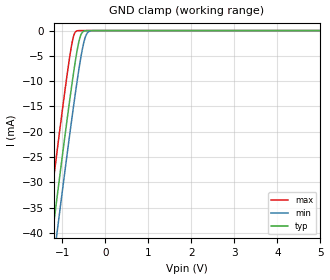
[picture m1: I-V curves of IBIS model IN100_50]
| TEXAS INSTRUMENTS INCORPORATED - Standard Linear and
|   Logic Group / High Volume Linear
| EMI Filter with Integrated VCC Clamp for SIM Card Interface
| Part#   VCC Voltage Range   Package-type   #pins
|TPD6F002QDSV   4.5 to 5.5V   QFN   13
[IBIS Ver]   3.2
[Comment char]  |_char
[File Name]   tpd6f002.ibs
[File Rev]   1.0 | A0
[Date]   December 10, 2014
[Source]   Data created from TI-SPICE simulations at TI-SLL/HVL.
   The following is an IBIS list for the TPD6F002.
   Please contact sllibis@ti.com with questions and
   comments concerning SLL IBIS models.
[Notes]   Revision History:
   1.0: 02/24/2011
   - Initial version of the model
   - This file contains package information for the SOT 8-pin
   (DSV) package as [Component] TPD6F002_DSV
   - This device can be powered at 5 volt Vcc
[Disclaimer]
| This model is designed as an aid for customers of Texas Instruments.
| TI and its licensors and suppliers make no warranties, either expressed
| or implied, with respect to this  model, including the warranties of
| merchantability or fitness for a particular purpose. The model is
| provided solely on an "as is" basis. The entire risk as to its quality
| and performance is with the customer.
[Copyright]
| (C) Copyright 2011 Texas Instruments Incorporated. All rights reserved.
| Component TPD6F002_DSV 13-PIN QFN
[Component]   TPD6F002_DSV
[Manufacturer]   Texas Instruments, Inc.
[Package]
|   typ   min   max
R_pkg   5.374e-02   1.500e-02   5.374e-02
L_pkg   6.554e-10   6.400e-12   7.112e-10
C_pkg   9.454e-14   5.280e-14   9.871e-14
[Pin]   signal_name   model_name   R_pin   L_pin   C_pin
1   Ch1_In   IN100_50   5.701e-02   7.112e-10   8.801e-14
2   Ch1_In   IN100_50   5.253e-02   6.367e-10   9.865e-14
3   Ch1_In   IN100_50   5.161e-02   6.235e-10   9.692e-14
4   Ch1_In   IN100_50   5.172e-02   6.216e-10   9.691e-14
5   Ch1_In   IN100_50   5.260e-02   6.372e-10   9.871e-14
6   Ch1_In   IN100_50   5.707e-02   7.096e-10   8.808e-14
7   Ch1_In   IN100_50   5.714e-02   7.049e-10   8.802e-14
8   Ch1_In   IN100_50   5.251e-02   6.347e-10   9.869e-14
9   Ch1_In   IN100_50   5.169e-02   6.178e-10   9.692e-14
10   Ch1_In   IN100_50   5.157e-02   6.226e-10   9.689e-14
11   Ch1_In   IN100_50   5.252e-02   6.375e-10   9.868e-14
12   Ch1_In   IN100_50   5.695e-02   7.074e-10   8.802e-14
13   GND   POWER   1.500e-02   6.400e-12   5.280e-14
| Models and submodels in the file (1): IN100_50 (Input)
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[Model]   IN100_50
Model_type  Input
Vinl=1.75
Vinh=3.25
| variable   typ   min   max
C_comp   34.0pF   23.8pF   44.2pF
[Temperature Range]   40   100   -40
| Ambient temperature   25   85   -40
[Voltage range]   5   4.5   5.5
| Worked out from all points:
|   GND clamp passes 1 mA (typ) near -0.57 V on its own axis
[GND Clamp]
| IN100_50
|   Voltage   I(typ)   I(min)   I(max)
-5V       -304.8mA   -311.4mA   -296.4mA
-1.35V    -48.74mA   -55.7mA    -39.68mA
-1.23V    -40.56mA   -47.53mA   -31.47mA
-1.13V    -33.79mA   -40.77mA   -24.71mA
-1.095V   -31.44mA   -38.42mA   -22.36mA
-800mV    -12.27mA   -19.04mA   -3.895mA
-730mV    -8.099mA   -14.67mA   -974.8uA
-665mV    -4.585mA   -10.76mA   -86.23uA
-580mV    -1.209mA   -6.047mA   -1.421uA
-495mV    -110.6uA   -2.294mA   -21.2nA
-350mV    -579.4nA   -83.81uA   -365.9pA
5V        5.011nA    6.712nA    5.01nA
